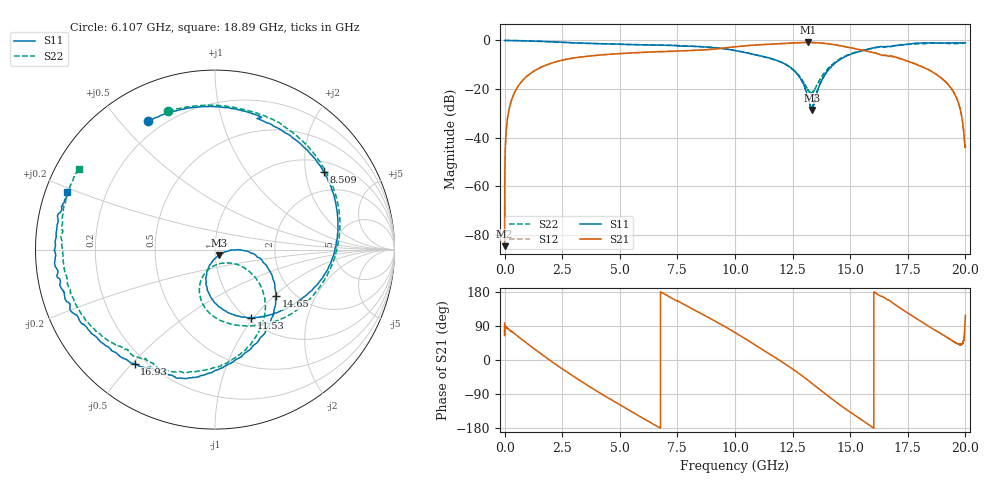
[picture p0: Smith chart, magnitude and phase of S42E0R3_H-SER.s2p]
!{S42E0R3}
!Johanson Technology Inc.
!www.johansontechnology.com
!Test Board Conditions:
!Substrate Type  RO4350B
!Substrate Thickness  50 mil
!Substrate Dk  3.66
!TL Type: GCPW
!TL Trace Width  60 mil
!TL Gap  10 mil
!Electrode orientation  Horizontal
!DUT TOPOLOGY	SERIES
!Mounting Pad LxW  14x55 mil
! Created Wed Nov 25 20:16:00 2020
# khz S ma R 50
! 2 Port Network Data from SP1.SP block
! freq  magS11  angS11  magS21  angS21  magS12  angS12  magS22  angS22
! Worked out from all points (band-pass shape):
!   20001 points, 300 kHz to 20 GHz, reference 50 ohm
!   highest |S21| = -0.82 dB at 13.17 GHz (marker M1); lowest = -84.8 dB at 300 kHz (marker M2)
!   |S21| within 3 dB of the highest: 8.749962 GHz to 8.752047 GHz (2.084 MHz wide, 0.0238 % of centre); 8.759 GHz to 15.41 GHz (6.653 GHz wide, 55.1 % of centre)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
!   lowest |S11| = -28.6 dB at 13.34 GHz (marker M3), VSWR 1.08, Z = 52.1 - j3.14 ohm
!   |S11| at or under -10 dB: 12.2251 GHz to 12.22708 GHz (1.974 MHz wide, 0.0161 % of centre); 12.23 GHz to 14.27 GHz (2.042 GHz wide, 15.4 % of centre); 14.27043 GHz to 14.27239 GHz (1.959 MHz wide, 0.0137 % of centre)
!   |S22| runs from -21.8 to 0.0 dB; largest |S21 - S12| = 0.017
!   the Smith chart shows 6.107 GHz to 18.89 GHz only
!   S11 on the Smith chart (normalised r, x): 6.107 GHz: 0.15, +0.59; 8.509 GHz: 1.29, +2.52; 11.53 GHz: 1.04, -0.97; 14.65 GHz: 1.62, -1.03; 16.93 GHz: 0.16, -0.51; 18.89 GHz: 0.07, +0.19
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300  0.9992 -0.3  5.76e-05 97.5  0.0001013 43.2  1 -0.3
139300  0.9995 -6.5  0.02732 82.9  0.02746 83.0  0.9987 -6.6
527300  0.9946 -25.0  0.1026 64.8  0.1029 65.0  0.9938 -25.5
1849300  0.9481 -84.8  0.3165 4.4  0.3179 4.4  0.9409 -86.4
3334300  0.881 -146.8  0.4576 -56.6  0.4576 -56.6  0.879 -146.1
4625300  0.8448 166.1  0.5219 -104.6  0.5218 -104.8  0.8475 165.3
6107300  0.8066 117.7  0.5752 -157.3  0.5719 -157.4  0.8142 108.6
6667300  0.8008 98.9  0.588 -176.7  0.5867 -176.9  0.8033 88.7
8509300  0.7447 35.7  0.6343 123.2  0.6327 123.1  0.7481 30.7
1.00003e7  0.6205 -14.1  0.7422 72.7  0.741 72.9  0.6223 -18.7
1.15313e7  0.4278 -62.2  0.8366 14.6  0.8395 14.7  0.4244 -77.8
1.25973e7  0.2314 -100.5  0.8924 -28.0  0.8948 -28.2  0.2335 -111.9
1.31653e7  0.06671 -102.4  0.9104 -53.4  0.907 -53.3  0.09635 -98.2
1.33343e7  0.03786 -56.7  0.9044 -61.4  0.9041 -61.3  0.08308 -69.4
1.33373e7  0.03702 -54.3  0.9037 -61.5  0.9041 -61.5  0.08295 -69.3
1.38873e7  0.1921 -4.1  0.8701 -87.5  0.8752 -87.4  0.2181 -32.6
1.46493e7  0.4273 -37.5  0.7635 -122.9  0.768 -122.6  0.442 -51.0
1.66673e7  0.7491 -117.6  0.4753 158.3  0.4635 158.6  0.7464 -129.7
1.69293e7  0.7773 -125.2  0.4608 146.9  0.4472 147.5  0.7781 -138.6
1.88853e7  0.8817 158.7  0.1778 71.3  0.1779 70.9  0.8808 149.4
1.96273e7  0.8995 132.2  0.06362 44.0  0.06446 43.6  0.8579 118.1
2e7  0.898 119.5  0.006462 117.6  0.006589 118.6  0.8764 98.3
